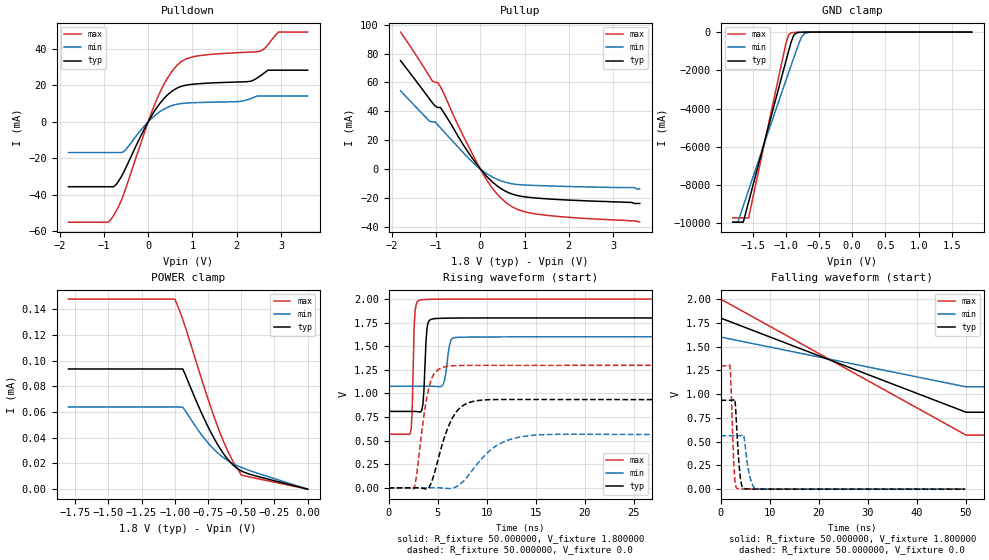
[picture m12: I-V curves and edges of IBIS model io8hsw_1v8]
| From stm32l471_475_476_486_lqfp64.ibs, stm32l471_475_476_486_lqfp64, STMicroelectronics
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|   Model io8hsw_1v8
[Model]  io8hsw_1v8
Model_type I/O
Polarity   Non-Inverting
Enable   Active-Low
Vinl =   0.540000V
Vinh =   1.260000V
Vmeas =  0.900000V
Cref =   100.000000nF
Rref =   1.000000k
Vref =   1.800000V
C_comp   3.002500pF   2.845500pF   3.023700pF
[Temperature Range]   25.000000   0.125000k   -40.000000
[Pullup Reference]   1.800000V   1.600000V   2.000000V
[Pulldown Reference]   0.0V   0.0V   0.0V
[POWER Clamp Reference]   1.800000V   1.600000V   2.000000V
[GND Clamp Reference]   0.0V   0.0V   0.0V
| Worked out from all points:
|   slope of the pulldown table from 0 to 0.27 V, typ, clamps not added: 26.4 ohm
|   slope of the pullup table from 0 to 0.27 V, typ, clamps not added: 30.1 ohm
|   GND clamp passes 1 mA (typ) near -0.58 V on its own axis
|   rising waveform, R_fixture 50.000000, V_fixture 1.800000: 20-80 % time 264ps typ, 404ps min, 196ps max; typ from 0.81 V to 1.8 V
|   rising waveform, R_fixture 50.000000, V_fixture 0.0: 20-80 % time 1.79ns typ, 3.05ns min, 1.06ns max; typ from 0.001 V to 0.935 V
|   falling waveform, R_fixture 50.000000, V_fixture 1.800000: 20-80 % time 30ns typ, 30ns min, 30ns max; typ from 1.8 V to 0.81 V
|   falling waveform, R_fixture 50.000000, V_fixture 0.0: 20-80 % time 719ps typ, 1.03ns min, 555ps max; typ from 0.935 V to 0.001 V
[Pulldown]
|Voltage   I(typ)   I(min)   I(max)
-1.8V     -35.64mA   -16.93mA   -55.1mA
-840mV    -35.64mA   -16.93mA   -53.52mA
-720mV    -34.31mA   -16.93mA   -48.86mA
-540mV    -27.04mA   -16.13mA   -38.89mA
240mV     9.303mA    5.14mA     14.78mA
480mV     15.67mA    8.374mA    25.64mA
720mV     19.18mA    9.883mA    32.46mA
1.14V     20.87mA    10.54mA    36.19mA
2.28V     22.08mA    12.36mA    38.18mA
2.52V     24.96mA    14.17mA    38.63mA
2.94V     28.28mA    14.17mA    49.19mA
3.6V      28.28mA    14.17mA    49.19mA
[Pullup]
|Voltage   I(typ)   I(min)   I(max)
-1.8V     75.08mA    54.18mA    94.95mA
-1.14V    48.3mA     32.94mA    63.91mA
-1.08V    45.81mA    32.62mA    60.91mA
-960mV    42.6mA     30.54mA    60.04mA
-900mV    42.6mA     28.5mA     57.07mA
-480mV    21.53mA    14.44mA    28.9mA
0V        40fA       141.7pA    0A
300mV     -9.801mA   -6.008mA   -14.46mA
600mV     -15.96mA   -9.582mA   -23.81mA
900mV     -18.89mA   -10.98mA   -28.81mA
1.32V     -20.37mA   -11.6mA    -31.56mA
3.6V      -24mA      -14mA      -37mA
[GND_clamp]
|Voltage   I(typ)   I(min)   I(max)
-1.8V     -9.93A     -9.932A    -9.707A
-1.72V    -9.93A     -9.932A    -9.707A
-1.64V    -9.93A     -9.083A    -9.707A
-1.56V    -8.876A    -8.251A    -9.707A
-1V       -1.54A     -2.541A    -631mA
-960mV    -1.028A    -2.139A    -153.7mA
-920mV    -527mA     -1.74A     -39.12mA
-880mV    -155.6mA   -1.344A    -18.01mA
-840mV    -45.32mA   -953mA     -12.68mA
-760mV    -8.418mA   -235mA     -7.62mA
-680mV    -3.44mA    -33.01mA   -3.865mA
1.8V      0A         0A         0A
[POWER_clamp]
|Voltage   I(typ)   I(min)   I(max)
-1.8V     93.65uA    63.98uA    148.1uA
-1V       93.65uA    63.98uA    148.1uA
-940mV    93.65uA    63.82uA    132.2uA
-780mV    55.19uA    39.85uA    79.88uA
-720mV    42.64uA    32.64uA    61.13uA
-680mV    35.2uA     28.59uA    49.56uA
-640mV    28.65uA    25.14uA    38.93uA
-600mV    23.11uA    22.24uA    29.46uA
-560mV    18.7uA     19.84uA    21.37uA
-500mV    14.28uA    16.96uA    11.08uA
-400mV    10.58uA    13.2uA     8.679uA
0V        0A         0A         0A
[Ramp]
| variable   typ   min   max
dV/dt_r  0.56073/1.79170n   0.33711/3.03795n   0.77863/1.05387n
dV/dt_f  0.59411/1.73150n   0.31410/3.03748n   0.85869/0.96383n
R_load = 50.000000
[Rising Waveform]
R_fixture= 50.000000
V_fixture= 1.800000
V_fixture_min= 1.600000
V_fixture_max= 2.000000
|time   V(typ)   V(min)   V(max)
0s        809.8mV    1.076V     568.8mV
2.202ns   809.8mV    1.076V     575.5mV
2.402ns   809.8mV    1.076V     805mV
2.703ns   809.5mV    1.076V     1.875V
3.203ns   803.9mV    1.077V     1.99V
3.504ns   893.5mV    1.077V     1.994V
3.904ns   1.681V     1.077V     1.996V
4.505ns   1.79V      1.076V     1.998V
6.907ns   1.799V     1.593V     2V
49.85ns   1.8V       1.6V       2V
[Rising Waveform]
R_fixture= 50.000000
V_fixture= 0.0
V_fixture_min= 0.0
V_fixture_max= 0.0
|time   V(typ)   V(min)   V(max)
0s        727.6uV    1.154mV    483.6uV
2.603ns   742.7uV    1.154mV    -6.412mV
4.104ns   4.724mV    1.159mV    1.059V
4.705ns   167mV      1.251mV    1.218V
5.506ns   472.8mV    -1.31mV    1.276V
6.507ns   740.7mV    -4.077mV   1.293V
7.708ns   879.9mV    80.01mV    1.297V
10.31ns   934.2mV    393.9mV    1.298V
13.51ns   936.5mV    542.3mV    1.298V
49.85ns   935.3mV    563.1mV    1.298V
[Falling Waveform]
R_fixture= 50.000000
V_fixture= 1.800000
V_fixture_min= 1.600000
V_fixture_max= 2.000000
|time   V(typ)   V(min)   V(max)
0s        1.8V       1.6V       2V
50.05ns   809.8mV    1.077V     568.9mV
150.2ns   809.8mV    1.076V     568.8mV
4.955us   809.8mV    1.076V     568.8mV
[Falling Waveform]
R_fixture= 50.000000
V_fixture= 0.0
V_fixture_min= 0.0
V_fixture_max= 0.0
|time   V(typ)   V(min)   V(max)
0s        935.3mV    563.1mV    1.298V
1.902ns   935.3mV    563.1mV    1.3V
2.803ns   948.9mV    563.1mV    157.6mV
3.403ns   522.9mV    562.9mV    6.336mV
3.904ns   172.9mV    562.7mV    2.713mV
4.304ns   37.82mV    567.8mV    1.95mV
4.705ns   9.576mV    562.4mV    1.572mV
5.906ns   2.082mV    140.3mV    1.025mV
7.207ns   1.26mV     7.648mV    833.2uV
49.85ns   727.6uV    1.154mV    483.6uV
